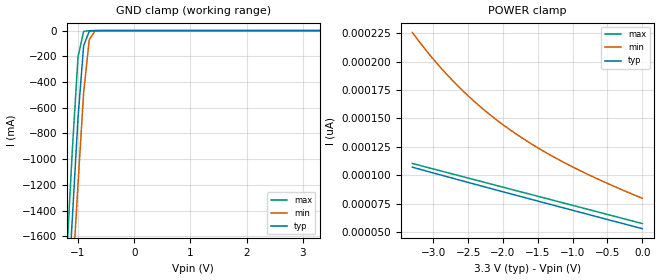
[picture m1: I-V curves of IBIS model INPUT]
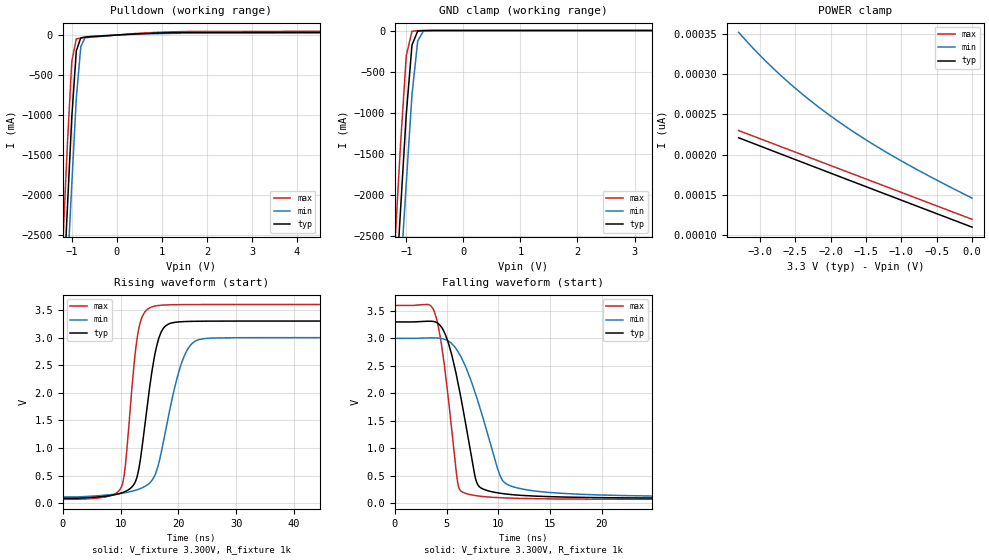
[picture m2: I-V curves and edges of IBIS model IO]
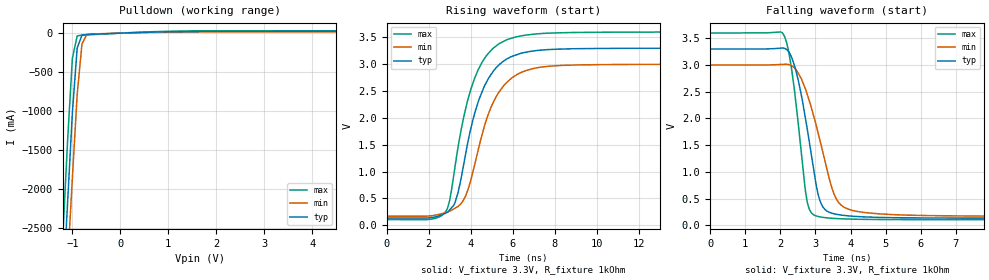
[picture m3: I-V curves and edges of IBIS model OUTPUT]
|   DIODES INCORPORATED
|   IBIS Model of PT7C4337
|   Product Family: 7C
|   8 Pin (W) SOIC Package
[IBIS Ver] 4.0
[Comment char] |_char
[File Name] pt7c4337_w_33v.ibs
[File Rev] 1.0
[Source] File originated at Diodes Incorporated.
[Date] 6/28/2018
[Disclaimer] (C) Copyright DIODES INCORPORATED
   All rights reserved
  Diodes Incorporated hereby grants the user of
  this IBIS model a non-exclusive, nontransferable license to
  use this IBIS model under the following terms.
  This IBIS model is provided on an "AS IS" basis and Diodes
  makes absolutely no warranty with respect to the information
  contained herein. DIODES DISCLAIMS AND CUSTOMER WAIVES ALL
  WARRANTIES, EXPRESSED OR IMPLIED, INCLUDING WARRANTIES OF
  MERCHANTABILITY OR FITNESS FOR A PARTICULAR PURPOSE. The
  entire risk as to quality and performance is with the customer.
  Accordingly, in no event shall the company be liable for any
  damages, whether in contract or tort, including any lost
  profits or other incidental, consequential, exemplary, or
  punitive damages arising out of the use or application of the
  IBIS model provided in this package. Further, Diodes reserves
  the right to make changes without notice to any product herein
  to improve reliability, function, or design. Diodes does not
  convey any license under patent rights or any other intellectual
  property rights, including those of third parties.
  The user is granted this license only to use the IBIS model
  and is not granted rights to sell, load, rent, lease or license
  the IBIS model in whole or in part, or in modified form to anyone
  other than user. User may modify the IBIS model to suit its specific
  application but rights to derivative works and such modifications
  shall belong to Diodes.
  Diodes is not obligated to provide maintenance or support
  for the licensed IBIS model.
  Contact Diodes at ATTN: APPLICATION ENGINEERING / IBIS MODELS
  1545 Barber Ln. Milpitas, CA 95035
[Component] PT7C4337
[Manufacturer] Diodes Incorporated.
[Package]
|   typ   min   max
R_pkg   0.03093ohm   0.02906ohm   0.03279ohm
L_pkg   2.23473nH   2.04677nH   2.42269nH
C_pkg   0.22955pF   0.20548pF   0.25361pF
[Pin]   signal_name   model_name   R_pin   L_pin   C_pin
1   X1   NC   0.03279   2.42269nH   0.25361pF
2   X2   NC   0.02906   2.04677nH   0.20548pF
3   _INTA   OUTPUT   0.02906   2.04677nH   0.20548pF
4   GND   GND   0.03279   2.26239nH   0.25361pF
5   SDA   IO   0.03279   2.42269nH   0.25361pF
6   SCL   INPUT   0.03279   2.42269nH   0.25361pF
7   SQW/_INTB   OUTPUT   0.02906   2.04677nH   0.20548pF
8   VCC   POWER   0.03279   2.42269nH   0.25361pF
| Models and submodels in the file (3): INPUT (Input), IO (I/O_open_drain), OUTPUT (Open_drain)
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|   Model INPUT1
[Model] INPUT
Model_type Input
Vinl = 990mV
Vinh = 2.31V
| variable   typ   min   max
C_comp   1.20pF   1.10pF   1.30pF
[Voltage Range]   3.30V   3.00V   3.60V
[GND Clamp Reference]   0.00V   0.00V   0.00V
[POWER Clamp Reference]  3.30V   3.00V   3.60V
[temperature range]   25   85   -40
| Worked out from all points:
|   GND clamp passes 1 mA (typ) near -0.71 V on its own axis
[GND Clamp]
| Voltage   I(typ)   I(min)  I(max)
-3.3V     -18.52A    -18.19A    -18.98A
-1.2V     -2.228A    -2.673A    -1.742A
-1.1V     -1.452A    -1.934A    -921.1mA
-1V       -678.8mA   -1.196A    -205.4mA
-900mV    -117.9mA   -482.7mA   -6.189mA
-800mV    -5.043mA   -71.03mA   -793.1uA
-700mV    -429.4uA   -4.115mA   -100.8uA
3.3V      53.12pA    87.55pA    52.8pA
[POWER Clamp]
| Voltage   I(typ)   I(min)  I(max)
-3.3V     107.2pA    225.7pA    110.4pA
-3V       102.1pA    202.1pA    105.6pA
-2.7V     97.09pA    181.8pA    100.8pA
-2.4V     92.11pA    164.3pA    96.01pA
-2.2V     88.81pA    154pA      92.8pA
-2V       85.53pA    144.5pA    89.61pA
-1.6V     79.01pA    127.9pA    83.21pA
-1.1V     70.87pA    110.5pA    75.2pA
-600mV    62.79pA    95.66pA    67.2pA
0V        53.11pA    79.85pA    57.6pA
|   Model IO
[Model]  IO
Model_type I/O_open_drain
Vinl = 990mV
Vinh = 2.31V
Vref=3.300V
Rref=1k
Vmeas=2.5V
| variable   typ   min   max
C_comp   1.184pF   1.183pF   1.185pF
[Voltage Range]   3.3000V   3.0000V   3.6000V
[POWER Clamp Reference]  3.3000V   3.0000V   3.6000V
[GND Clamp Reference]   0.0000V   0.0000V   0.0000V
[Pulldown Reference]   0.0000V   0.0000V   0.0000V
[Temperature Range]   25   85   -40
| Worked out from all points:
|   slope of the pulldown table from 0 to 0.495 V, typ, clamps not added: 32.1 ohm
|   GND clamp passes 1 mA (typ) near -0.70 V on its own axis
|   rising waveform, V_fixture 3.300V, R_fixture 1k: 20-80 % time 2.53ns typ, 3.67ns min, 1.82ns max; typ from 0.089 V to 3.3 V
|   falling waveform, V_fixture 3.300V, R_fixture 1k: 20-80 % time 1.94ns typ, 2.85ns min, 1.31ns max; typ from 3.3 V to 0.089 V
[GND Clamp]
| Voltage   I(typ)   I(min)  I(max)
-3.3V     -27.79A    -27.24A    -28.47A
-1.2V     -3.342A    -4.065A    -2.613A
-1.1V     -2.178A    -2.961A    -1.382A
-1V       -1.018A    -1.858A    -308mA
-900mV    -176.7mA   -782.5mA   -9.228mA
-800mV    -7.547mA   -127.2mA   -1.241mA
-700mV    -671uA     -7.764mA   -169.9uA
-500mV    -5.404uA   -45.45uA   -274.6nA
3.3V      110.2pA    159.5pA    109.9pA
[POWER Clamp]
| Voltage   I(typ)   I(min)  I(max)
-3.3V     221pA      351.5pA    229.9pA
-3V       210.8pA    323.2pA    219.9pA
-2.6V     197.3pA    290pA      206.5pA
-2.3V     187.2pA    267.9pA    196.5pA
-1.9V     173.8pA    241.7pA    183.2pA
-1.5V     160.4pA    218.4pA    169.9pA
-1.1V     147pA      197.3pA    156.6pA
-600mV    130.3pA    173.1pA    139.9pA
0V        110.2pA    146.2pA    119.9pA
[Pulldown]
| Voltage   I(typ)   I(min)  I(max)
-3.3V     -27.8A     -27.25A    -28.48A
-1.2V     -3.35A     -4.071A    -2.622A
-1.1V     -2.186A    -2.968A    -1.391A
-1V       -1.027A    -1.864A    -331.5mA
-900mV    -198.6mA   -791.1mA   -49.01mA
-800mV    -35.08mA   -143.9mA   -38.17mA
-700mV    -25.59mA   -26.1mA    -33.22mA
400mV     12.92mA    9.236mA    17.95mA
1.3V      29.49mA    20.96mA    40.83mA
6.6V      42.5mA     30.36mA    58.25mA
[Rising Waveform]
V_fixture = 3.300V
V_fixture_min = 3.00V
V_fixture_max = 3.600V
R_fixture = 1k
|   Time   V(typ)   V(min)   V(max)
0s        88.67mV    112.6mV    69.39mV
10.2ns    185.4mV    179.4mV    309.9mV
10.8ns    210.4mV    189.9mV    660.7mV
13ns      544.3mV    247.5mV    3.085V
15ns      2.086V     364.2mV    3.539V
16.2ns    2.832V     581.9mV    3.577V
17.4ns    3.17V      1.113V     3.59V
20.4ns    3.288V     2.496V     3.598V
23ns      3.296V     2.942V     3.599V
60ns      3.3V       3V         3.6V
[Falling Waveform]
V_fixture = 3.300V
V_fixture_min = 3.00V
V_fixture_max = 3.600V
R_fixture = 1k
|   Time   V(typ)   V(min)   V(max)
0s        3.3V       3V         3.6V
3.5ns     3.313V     3.01V      3.588V
4ns       3.293V     3.008V     3.377V
4.6ns     3.178V     2.995V     2.757V
6.2ns     2.093V     2.726V     270.7mV
7.8ns     437.5mV    1.982V     136.9mV
8.6ns     250.2mV    1.495V     118.7mV
10.7ns    166.8mV    358.7mV    94.5mV
18.5ns    103.3mV    156.9mV    72.86mV
201ns     88.67mV    112.6mV    69.39mV
[Ramp]
| variable   typ   min   max
dV/dt_r   1.9259V/2.5229n   1.7306V/3.5900n   2.1177V/1.8163n
dV/dt_f   1.9259V/1.9428n   1.7306V/2.8297n   2.1177V/1.3133n
R_load = 1000
|   Model OUTPUT
[Model]  OUTPUT
Model_type Open_drain
Vref = 3.30V
Rref = 1k
Cref =  0
Vmeas = 1.65V
| variable   typ   min   max
C_comp   1.361pF   1.358pF   1.364pF
[Voltage Range]   3.3000V   3.0000V   3.6000V
[POWER Clamp Reference]  3.3000V   3.0000V   3.6000V
[GND Clamp Reference]   0.0000V   0.0000V   0.0000V
[Pullup Reference]   3.3000V   3.0000V   3.6000V
[Pulldown Reference]   0.0000V   0.0000V   0.0000V
[Temperature Range]   25   85   -40
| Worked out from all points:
|   slope of the pulldown table from 0 to 0.495 V, typ, clamps not added: 48.1 ohm
|   rising waveform, V_fixture 3.3V, R_fixture 1kOhm: 20-80 % time 1.26ns typ, 1.34ns min, 1.22ns max; typ from 0.133 V to 3.3 V
|   falling waveform, V_fixture 3.3V, R_fixture 1kOhm: 20-80 % time 491ps typ, 678ps min, 360ps max; typ from 3.3 V to 0.133 V
[Pulldown]
|Voltage   I(typ)   I(min)   I(max)
-3.3V     -27.79A    -27.25A    -28.48A
-1.2V     -3.347A    -4.069A    -2.619A
-1.1V     -2.183A    -2.966A    -1.388A
-1V       -1.024A    -1.862A    -323.7mA
-900mV    -191.3mA   -788.3mA   -35.75mA
-800mV    -25.9mA    -138.3mA   -25.86mA
-700mV    -17.29mA   -19.99mA   -22.2mA
100mV     2.404mA    1.717mA    3.353mA
1.3V      19.66mA    13.98mA    27.22mA
6.6V      28.33mA    20.24mA    38.83mA
[Rising Waveform]
V_fixture = 3.3V
V_fixture_min = 3.0V
V_fixture_max = 3.6V
R_fixture = 1kOhm
C_fixture = 0F
|   Time   V(typ)   V(min)   V(max)
0s        133.3mV    169mV      104.4mV
2.8ns     223mV      233.7mV    248.2mV
3ns       284.5mV    259.6mV    458.4mV
3.4ns     606.6mV    349.7mV    1.455V
3.85ns    1.517V     639mV      2.315V
4.35ns    2.288V     1.39V      2.891V
5.2ns     2.928V     2.387V     3.336V
6.5ns     3.213V     2.862V     3.535V
10.3ns    3.293V     2.992V     3.595V
51ns      3.3V       3V         3.6V
[Falling Waveform]
V_fixture = 3.3V
V_fixture_min = 3.0V
V_fixture_max = 3.6V
R_fixture = 1kOhm
C_fixture = 0F
|   Time   V(typ)   V(min)   V(max)
0s        3.3V       3V         3.6V
2.08ns    3.318V     3.015V     3.582V
2.32ns    3.145V     2.986V     2.924V
2.78ns    1.744V     2.422V     395.3mV
3.08ns    568.7mV    1.716V     163.6mV
3.32ns    270.7mV    1.068V     138.9mV
3.54ns    213.3mV    567.1mV    127.8mV
3.82ns    183.5mV    335.5mV    119mV
5.6ns     138.9mV    189.9mV    105.6mV
51ns      133.3mV    169mV      104.4mV
[Ramp]
| variable   typ   min   max
dV/dt_r  1.9001V/1.2647n   1.7003V/1.3475n   2.0972V/1.2220n
dV/dt_f  1.9001V/498.88p   1.7003V/672.96p   2.0972V/362.48p
R_load = 1000
